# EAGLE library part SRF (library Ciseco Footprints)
SRF Wireless UART Serial Data Module. www.ciseco.co.uk
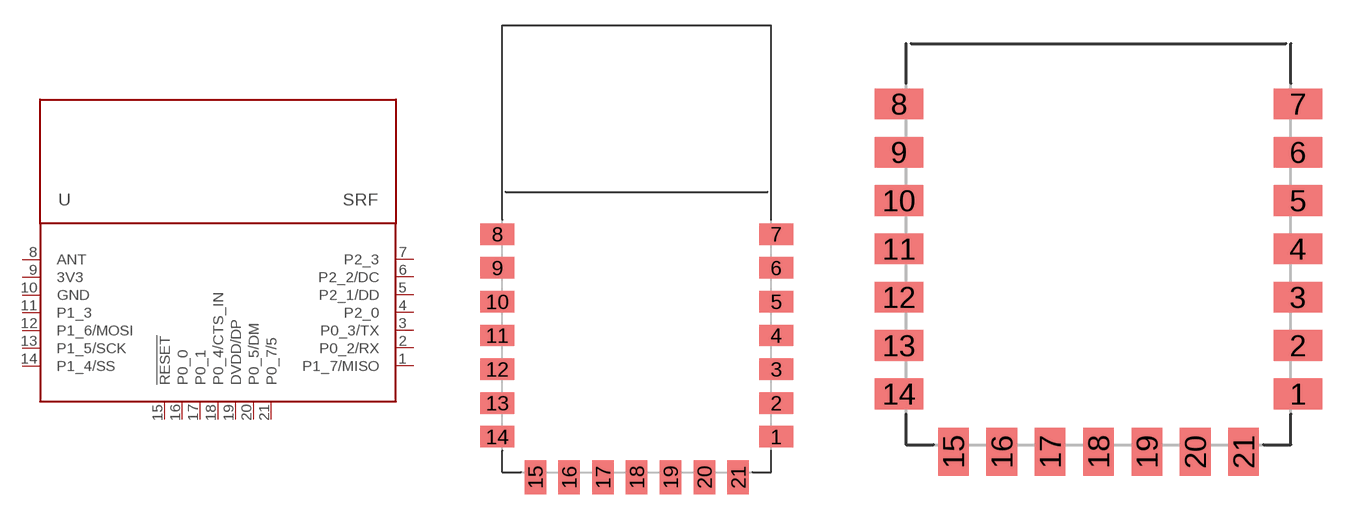
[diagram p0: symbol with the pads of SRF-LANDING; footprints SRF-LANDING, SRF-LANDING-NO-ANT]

Designator prefix U

## SRF-LANDING  [SRF-LANDING]
1  P1_7/MISO
2  P0_2/RX
3  P0_3/TX
4  P2_0
5  P2_1/DD
6  P2_2/DC
7  P2_3
8  ANT  out
9  3V3  pwr
10  GND  pwr
11  P1_3
12  P1_6/MOSI
13  P1_5/SCK
14  P1_4/SS
15  !RESET  in
16  P0_0
17  P0_1
18  P0_4/CTS_IN
19  DVDD/DP
20  P0_5/DM
21  P0_7/5

## SRF-LANDING-NO-ANT  [SRF-LANDING-NO-ANT]
Pads as for SRF-LANDING

## SRF-LANDING-1.0A  [SRF-LANDING-1.0A]
Pads as for SRF-LANDING

## SRF-LANDING-1.0A-MOVE  [SRF-LANDING-1.0A-MOVE]
Pads as for SRF-LANDING

## SRF-LANDING-NO-ANT-1.0A  [SRF-LANDING-NO-ANT-1.0A]
Pads as for SRF-LANDING

## SRF-LANDING-NO-ANT-1.0A-MOVE  [SRF-LANDING-NO-ANT-1.0A-MOVE]
Pads as for SRF-LANDING

## SRF-LANDING-1.2  [SRF-LANDING-1.2]
Pads as for SRF-LANDING

## SRF-LANDING-NO-ANT-1.2  [SRF-LANDING-NO-ANT-1.2]
Pads as for SRF-LANDING

## Footprint SRF-LANDING (pad centres in mm)
smd 2 x 1.27: 1 16.2,2; 2 16.2,4; 3 16.2,6; 4 16.2,8; 5 16.2,10; 6 16.2,12; 7 16.2,14; 8 -0.3,14; 9 -0.3,12; 10 -0.3,10; 11 -0.3,8; 12 -0.3,6; 13 -0.3,4; 14 -0.3,2
smd 1.27 x 2: 15 1.95,-0.4; 16 3.95,-0.4; 17 5.95,-0.4; 18 7.95,-0.4; 19 9.95,-0.4; 20 11.95,-0.4; 21 13.95,-0.4

## Footprint SRF-LANDING-NO-ANT (pad centres in mm)
smd 2 x 1.27: 1 16.2,2; 2 16.2,4; 3 16.2,6; 4 16.2,8; 5 16.2,10; 6 16.2,12; 7 16.2,14; 8 -0.3,14; 9 -0.3,12; 10 -0.3,10; 11 -0.3,8; 12 -0.3,6; 13 -0.3,4; 14 -0.3,2
smd 1.27 x 2: 15 1.95,-0.4; 16 3.95,-0.4; 17 5.95,-0.4; 18 7.95,-0.4; 19 9.95,-0.4; 20 11.95,-0.4; 21 13.95,-0.4

## Footprint SRF-LANDING-1.0A (pad centres in mm)
smd 2 x 1.27: 1 16.2,2; 2 16.2,4; 3 16.2,6; 4 16.2,8; 5 16.2,10; 6 16.2,12; 7 16.2,14; 8 -0.3,14; 9 -0.3,12; 10 -0.3,10; 11 -0.3,8; 12 -0.3,6; 13 -0.3,4; 14 -0.3,2
smd 1.27 x 2: 15 1.95,-0.4; 16 3.95,-0.4; 17 5.95,-0.4; 18 7.95,-0.4; 19 9.95,-0.4; 20 11.95,-0.4; 21 13.95,-0.4

## Footprint SRF-LANDING-1.0A-MOVE (pad centres in mm)
smd 2 x 1.27: 1 15.9,2; 2 15.9,4; 3 15.9,6; 4 15.9,8; 5 15.9,10; 6 15.9,12; 7 15.9,14; 8 0,14; 9 0,12; 10 0,10; 11 0,8; 12 0,6; 13 0,4; 14 0,2
smd 1.27 x 2: 15 1.95,-0.1; 16 3.95,-0.1; 17 5.95,-0.1; 18 7.95,-0.1; 19 9.95,-0.1; 20 11.95,-0.1; 21 13.95,-0.1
